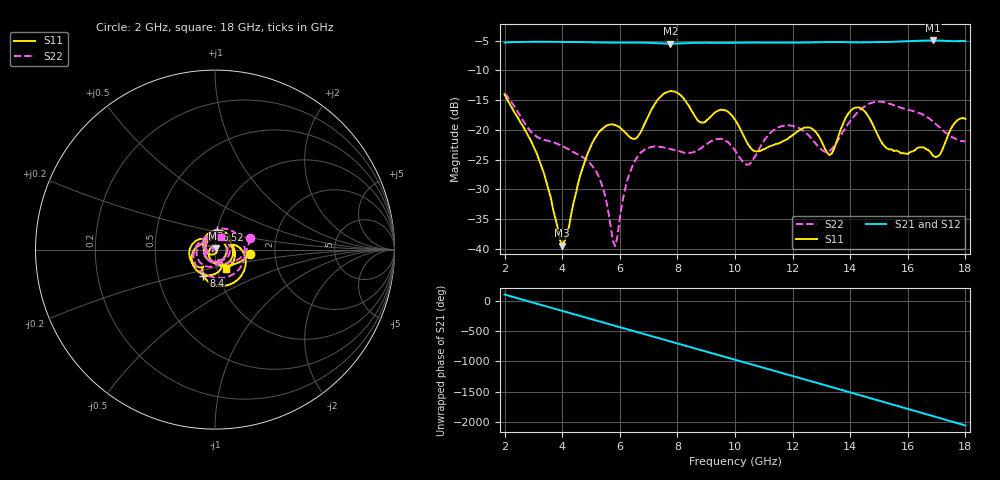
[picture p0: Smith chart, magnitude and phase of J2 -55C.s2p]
!Agilent Technologies,E8363B,SG43030131,A.07.50.48
!Agilent E8363B: A.07.50.48
!Date: Wednesday, December 17, 2025 22:26:26
!Correction: S11(Full 2 Port(1,2))
!S21(Full 2 Port(1,2))
!S12(Full 2 Port(1,2))
!S22(Full 2 Port(1,2))
!S2P File: Measurements: S11, S21, S12, S22:
# Hz S  dB  R 50
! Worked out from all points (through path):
!   201 points, 2 GHz to 18 GHz, reference 50 ohm
!   highest |S21| = -4.96 dB at 16.88 GHz (marker M1); lowest = -5.5 dB at 7.76 GHz (marker M2)
!   group delay of S21, straight-line fit = 373 ps
!   lowest |S11| = -39.4 dB at 4 GHz (marker M3), VSWR 1.02, Z = 50.7 + j0.807 ohm
!   |S11| at or under -10 dB: start of sweep to end of sweep
!   |S22| runs from -39.5 to -13.9 dB; largest |S21 - S12| = 0.0021
!   S11 on the Smith chart (normalised r, x): 2 GHz: 1.49, -0.07; 5.52 GHz: 1.00, +0.22; 8.4 GHz: 0.84, -0.25; 18 GHz: 1.10, -0.24
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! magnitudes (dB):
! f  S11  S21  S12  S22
! 2 GHz  -14.0  -5.3  -5.3  -13.9
! 3.12 GHz  -24.0  -5.2  -5.2  -21.2
! 4 GHz  -39.4  -5.2  -5.2  -22.7
! 4.72 GHz  -26.2  -5.2  -5.2  -24.6
! 5.52 GHz  -19.3  -5.3  -5.3  -31.7
! 5.84 GHz  -19.2  -5.3  -5.3  -39.5
! 6.4 GHz  -21.4  -5.3  -5.3  -26.5
! 7.36 GHz  -14.7  -5.4  -5.5  -22.8
! 7.76 GHz  -13.5  -5.5  -5.5  -23.2
! 8.4 GHz  -16.0  -5.4  -5.4  -23.9
! 8.8 GHz  -18.7  -5.3  -5.3  -23.1
! 10 GHz  -18.3  -5.3  -5.3  -23.4
! 10.4 GHz  -22.0  -5.3  -5.3  -25.8
! 10.72 GHz  -23.6  -5.3  -5.3  -24.3
! 11.6 GHz  -22.1  -5.3  -5.3  -19.4
! 12.72 GHz  -20.0  -5.3  -5.3  -21.8
! 13.28 GHz  -24.2  -5.2  -5.2  -23.5
! 13.92 GHz  -17.3  -5.3  -5.3  -19.0
! 14.32 GHz  -16.2  -5.3  -5.3  -16.8
! 15.36 GHz  -23.3  -5.2  -5.2  -15.6
! 16.88 GHz  -24.4  -5.0  -5.0  -18.6
! 18 GHz  -18.1  -5.1  -5.1  -21.9
